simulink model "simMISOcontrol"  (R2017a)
settings: Solver=VariableStepAuto  StartTime=0.0  StopTime=150  RelTol=1e-3
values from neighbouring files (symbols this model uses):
  step_d1 = -2.5    [MISOcontrol.m]    (also in MISO_demo.m; SISOcontrol.m = -2; init.m = 0)
  step_d2 = +2.5    (= 2.5)    [MISOcontrol.m]    (also in MISO_demo.m; SISOcontrol.m = 2; init.m = 0)
  step_ys1 = 5    [MISOcontrol.m]    (also in MISO_demo.m; SISOcontrol.m = 4)
  step_ys2 = -5    [MISOcontrol.m]    (also in MISO_demo.m; SISOcontrol.m = -4)
  stepTime_d1 = 90    [MISOcontrol.m]    (also in MISO_demo.m; SISOcontrol.m = 6; init.m = 0)
  stepTime_d2 = 120    [MISOcontrol.m]    (also in MISO_demo.m; SISOcontrol.m = 8; init.m = 0)
  stepTime_ys1 = 30    [MISOcontrol.m]
  stepTime_ys2 = 60    [MISOcontrol.m]
  sys_den11 = cell2mat(sys_tf11.den)    [MISOcontrol.m]    (also in MISO_demo.m; MIMOcontrol.m = cell2mat(sys_tf12.den))
  sys_den21 = cell2mat(sys_tf21.den)    [MISOcontrol.m]    (also in MISO_demo.m; MIMOcontrol.m = cell2mat(sys_tf32.den))
  sys_num11 = cell2mat(sys_tf11.num)    [MISOcontrol.m]    (also in MISO_demo.m; MIMOcontrol.m = cell2mat(sys_tf12.num))
  sys_num21 = cell2mat(sys_tf21.num)    [MISOcontrol.m]    (also in MISO_demo.m; MIMOcontrol.m = cell2mat(sys_tf32.num))
  Ts = 0.1    [identification.m]    (also in MISOcontrol.m; MISO_demo.m; runSteptest.m; SISOcontrol.m)
  y_s0 = 0    [MISOcontrol.m]    (also in MISO_demo.m; SISOcontrol.m = 4)
undefined symbols (not defined in the file or in its folder): Kb, Kc11, Kc21, tauI11, tauI21
libraries: simulink x2

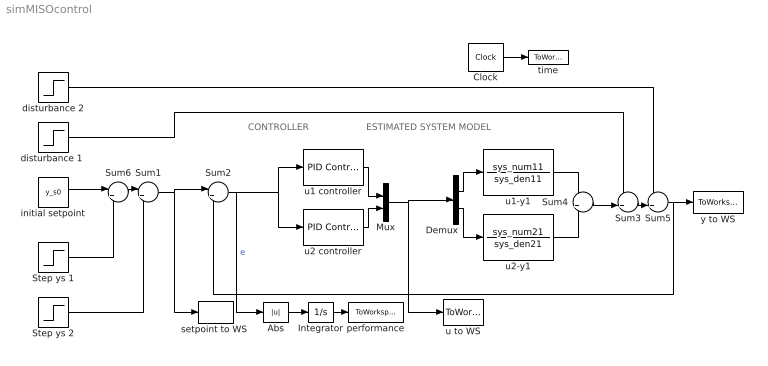
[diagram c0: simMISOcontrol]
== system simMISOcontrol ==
  note: ESTIMATED SYSTEM MODEL
  note: CONTROLLER
  Abs : Abs  ZeroCross=off
  Clock : Clock
  Demux : Demux  Outputs=2
  Integrator : Integrator  ZeroCross=off
  Mux : Mux  Inputs=2
  Step ys 1 : Step  Time=stepTime_ys1  After=step_ys1  SampleTime=Ts  ZeroCross=off
  Step ys 2 : Step  Time=stepTime_ys2  After=step_ys2  SampleTime=Ts  ZeroCross=off
  Sum1 : Sum  Inputs=|++
  Sum2 : Sum  Inputs=|+-
  Sum3 : Sum  Inputs=++|
  Sum4 : Sum
  Sum5 : Sum  Inputs=++|
  Sum6 : Sum  Inputs=|++
  "disturbance 1 " : Step  Time=stepTime_d1  After=step_d1  SampleTime=Ts  ZeroCross=off
  disturbance 2 : Step  Time=stepTime_d2  After=step_d2  SampleTime=Ts  ZeroCross=off
  initial setpoint : Constant  Value=y_s0  SampleTime=Ts
  performance : ToWorkspace  VariableName=IAE  SampleTime=Ts
  "setpoint to WS " : ToWorkspace  VariableName=ys  SampleTime=Ts
  time : ToWorkspace  VariableName=time  SampleTime=Ts
  u to WS : ToWorkspace  VariableName=u  SampleTime=Ts
  u1 controller : simulink/Continuous/PID Controller  Controller=PI  TimeDomain=Continuous-time  SampleTime=-1  IntegratorMethod=Forward Euler  FilterMethod=Forward Euler  Form=Parallel  UseFilter=on  ControllerParametersSource=internal  P=Kc11  I=Kc11/tauI11  D=0  N=100  InitialConditionSource=internal  InitialConditionForIntegrator=0  InitialConditionForFilter=0  ExternalReset=none  LimitOutput=on  UpperSaturationLimit=1  LowerSaturationLimit=0  LinearizeAsGain=on  AntiWindupMode=clamping  Kb=Kb  TrackingMode=off  Kt=1  PParamMin=[]  PParamMax=[]  IParamMin=[]  IParamMax=[]  DParamMin=[]  DParamMax=[]  NParamMin=[]  NParamMax=[]  KbParamMin=[]  KbParamMax=[]  KtParamMin=[]  KtParamMax=[]  POutMin=[]  POutMax=[]  IOutMin=[]  IOutMax=[]  DOutMin=[]  DOutMax=[]  NOutMin=[]  NOutMax=[]  KbOutMin=[]  KbOutMax=[]  KtOutMin=[]  KtOutMax=[]  IntegratorOutMin=[]  IntegratorOutMax=[]  FilterOutMin=[]  FilterOutMax=[]  SumOutMin=[]  SumOutMax=[]  SumI1OutMin=[]  SumI1OutMax=[]  SumI2OutMin=[]  SumI2OutMax=[]  SumI3OutMin=[]  SumI3OutMax=[]  SumDOutMin=[]  SumDOutMax=[]  SaturationOutMin=[]  SaturationOutMax=[]  IntegratorContinuousStateAttributes=''  IntegratorStateMustResolveToSignalObject=off  IntegratorRTWStateStorageClass=Auto  FilterContinuousStateAttributes=''  FilterStateMustResolveToSignalObject=off  FilterRTWStateStorageClass=Auto  DifferentiatorICPrevScaledInput=0  DifferentiatorOutMin=[]  DifferentiatorOutMax=[]  InitialConditionSetting=State (most efficient)
  u1-y1 : TransferFcn  Numerator=sys_num11  Denominator=sys_den11
  u2 controller : simulink/Continuous/PID Controller  Controller=PI  TimeDomain=Continuous-time  SampleTime=-1  IntegratorMethod=Forward Euler  FilterMethod=Forward Euler  Form=Parallel  UseFilter=on  ControllerParametersSource=internal  P=Kc21  I=Kc21/tauI21  D=0  N=100  InitialConditionSource=internal  InitialConditionForIntegrator=0  InitialConditionForFilter=0  ExternalReset=none  LimitOutput=on  UpperSaturationLimit=1  LowerSaturationLimit=0  LinearizeAsGain=on  AntiWindupMode=clamping  Kb=Kb  TrackingMode=off  Kt=1  PParamMin=[]  PParamMax=[]  IParamMin=[]  IParamMax=[]  DParamMin=[]  DParamMax=[]  NParamMin=[]  NParamMax=[]  KbParamMin=[]  KbParamMax=[]  KtParamMin=[]  KtParamMax=[]  POutMin=[]  POutMax=[]  IOutMin=[]  IOutMax=[]  DOutMin=[]  DOutMax=[]  NOutMin=[]  NOutMax=[]  KbOutMin=[]  KbOutMax=[]  KtOutMin=[]  KtOutMax=[]  IntegratorOutMin=[]  IntegratorOutMax=[]  FilterOutMin=[]  FilterOutMax=[]  SumOutMin=[]  SumOutMax=[]  SumI1OutMin=[]  SumI1OutMax=[]  SumI2OutMin=[]  SumI2OutMax=[]  SumI3OutMin=[]  SumI3OutMax=[]  SumDOutMin=[]  SumDOutMax=[]  SaturationOutMin=[]  SaturationOutMax=[]  IntegratorContinuousStateAttributes=''  IntegratorStateMustResolveToSignalObject=off  IntegratorRTWStateStorageClass=Auto  FilterContinuousStateAttributes=''  FilterStateMustResolveToSignalObject=off  FilterRTWStateStorageClass=Auto  DifferentiatorICPrevScaledInput=0  DifferentiatorOutMin=[]  DifferentiatorOutMax=[]  InitialConditionSetting=State (most efficient)
  u2-y1 : TransferFcn  Numerator=sys_num21  Denominator=sys_den21
  y to WS : ToWorkspace  VariableName=y  SampleTime=Ts
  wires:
  Clock/1 -> time/1
  Sum1/1 -> Sum2/1, "setpoint to WS "/1
  Sum3/1 -> Sum5/2
  Sum2/1 -> u2 controller/1, u1 controller/1, Abs/1  "e"
  Integrator/1 -> performance/1
  Abs/1 -> Integrator/1
  "disturbance 1 "/1 -> Sum3/1
  Sum5/1 -> y to WS/1, Sum2/2
  disturbance 2/1 -> Sum5/1
  u2-y1/1 -> Sum4/2
  Sum4/1 -> Sum3/2
  u1-y1/1 -> Sum4/1
  Demux/1 -> u1-y1/1
  Demux/2 -> u2-y1/1
  u1 controller/1 -> Mux/1
  u2 controller/1 -> Mux/2
  Mux/1 -> u to WS/1, Demux/1
  initial setpoint/1 -> Sum6/1
  Step ys 2/1 -> Sum1/2
  Sum6/1 -> Sum1/1
  Step ys 1/1 -> Sum6/2
